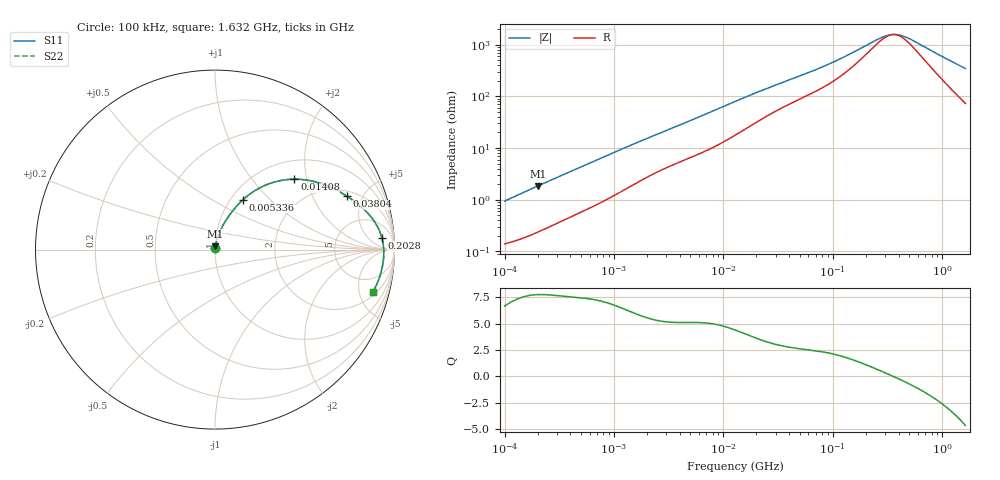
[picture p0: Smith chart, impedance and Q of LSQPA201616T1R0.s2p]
! LSQPA201616T1R0  S-PARAMETER MODEL  ( General Type )
! Model Generated by TAIYO YUDEN Corporation (http://www.ty-top.com)
! Version 2.0
! TAIYO YUDEN Control No. 100810NF25SB-FKC
! Copyright(c) 2007 TAIYO YUDEN CO.,LTD. All Rights Reserved.
! Product Description (link to TY-COMPAS)
! https://ds.yuden.co.jp/TYCOMPAS/or/detail?pn=LSQPA201616T1R0M&u=M
! Products Name : Inductors
! Characteristics :
!  Inductance : 1.0 uH , SRF(min) : 100 MHz , DC Resistance(max) : 0.13 Ohm
!  Rated Current : Saturation :1100 mA , Temp Rise : 1100 mA (40 degC)
!  Case Size : 2.0 x 1.6 / 0.079 x 0.063 [mm/inch] , Thickness : 1.6 / 0.063 [mm/inch]
!  (Conditions: Temperature = 25 degC , DC Bias Current/Voltage = 0A / 0V)
! External Node Assignments :
!  1  o---GGG---o  2
! GND o---------o GND
! Frequency Range : 0.1MHz  -  1631.998593MHz  [ 402 STEP ]
# MHz S RI R 50
! Freq[MHz].  S11 Real  S11 Imag  S21 Real  S21 Imag  S12 Real  S12 Imag  S22 Real  S22 Imag
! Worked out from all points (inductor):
!   401 points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, 100 kHz to 1.632 GHz, reference 50 ohm
!   read as one part in series: L = 1.48 uH near 105 kHz
!   highest Q = 7.75 at 202 kHz (marker M1), where L = 1.45 uH
!   self-resonance near 356.9 MHz
!   S11 on the Smith chart (normalised r, x): 100 kHz: 1.00, +0.02; 5.336 MHz: 1.14, +0.71; 14.08 MHz: 1.40, +1.69; 38.04 MHz: 2.33, +3.74; 202.8 MHz: 14, +14; 1.632 GHz: 2.45, -6.75
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0.1  0.00148 0.0093  0.9985 -0.0093  0.9985 -0.0093  0.00148 0.0093
0.202033  0.00271 0.0183  0.9973 -0.0183  0.9973 -0.0183  0.00271 0.0183
0.507727  0.00765 0.0428  0.9923 -0.0428  0.9923 -0.0428  0.00765 0.0428
1.186434  0.023 0.0914  0.977 -0.0914  0.977 -0.0914  0.023 0.0914
2.577871  0.0651 0.1695  0.9349 -0.1695  0.9349 -0.1695  0.0651 0.1695
3.79988  0.1045 0.2232  0.8955 -0.2232  0.8955 -0.2232  0.1045 0.2232
5.335991  0.1567 0.2786  0.8433 -0.2786  0.8433 -0.2786  0.1567 0.2786
8.058528  0.2541 0.3463  0.7459 -0.3463  0.7459 -0.3463  0.2541 0.3463
13.08855  0.4159 0.3913  0.5841 -0.3913  0.5841 -0.3913  0.4159 0.3913
14.07625  0.4422 0.3923  0.5578 -0.3923  0.5578 -0.3923  0.4422 0.3923
17.93928  0.5281 0.3847  0.4719 -0.3847  0.4719 -0.3847  0.5281 0.3847
23.42367  0.6132 0.3605  0.3868 -0.3605  0.3868 -0.3605  0.6132 0.3605
38.04441  0.7345 0.2979  0.2655 -0.2979  0.2655 -0.2979  0.7345 0.2979
64.86202  0.8305 0.2237  0.1695 -0.2237  0.1695 -0.2237  0.8305 0.2237
113.2979  0.8966 0.1435  0.1034 -0.1435  0.1034 -0.1435  0.8966 0.1435
202.7613  0.9299 0.0661  0.0701 -0.0661  0.0701 -0.0661  0.9299 0.0661
271.248  0.937 0.0314  0.063 -0.0314  0.063 -0.0314  0.937 0.0314
329.3222  0.9395 0.00918  0.0605 -0.00918  0.0605 -0.00918  0.9395 0.00918
390.2506  0.9404 -0.0102  0.0596 0.0102  0.0596 0.0102  0.9404 -0.0102
473.8032  0.9401 -0.0329  0.0599 0.0329  0.0599 0.0329  0.9401 -0.0329
957.2386  0.924 -0.1306  0.076 0.1306  0.076 0.1306  0.924 -0.1306
1631.999  0.88 -0.2348  0.12 0.2348  0.12 0.2348  0.88 -0.2348
